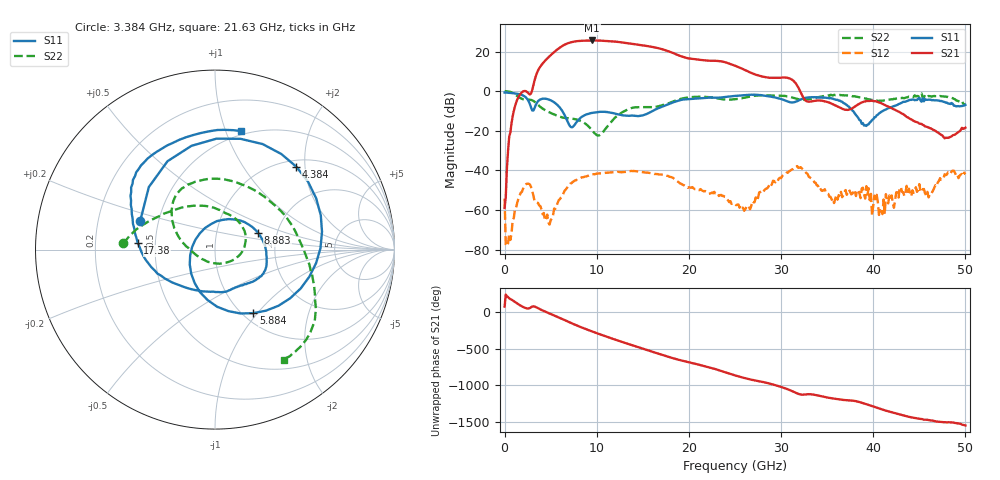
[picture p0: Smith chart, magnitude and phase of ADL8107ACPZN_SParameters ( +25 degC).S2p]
! Analog Devices, Inc.
! Device:	ADL8107ACPZN
! Description:	"GaAs, pHEMT, MMIC, Low Phase Noise Amplifier, 6 GHz to 18 GHz"
! Conditions:	Vdd = 5.0 V
!		IDQ = 90 mA quiescent (Self-biased mode)
!		Pin = -20 dBm
!		Operating Temperature = +25 C (at package bottom)
! Product validation unit SN7 soldered down to Evaluation Board as shown on ADL8107-EVALZ User Guide. Board loss de-embedded from S21 magnitude.  All other RF measurements reference to RF coaxial connector.
! Frequency (GHz)	S11_Mag (dB)	S11_Phase (deg)	S21_Mag (dB)	S21_Phase (deg)	S12_Mag (dB)	S12_Phase (deg)	S22_Mag (dB)	S22_Phase (deg)
#  GHZ  S  DB  R 50
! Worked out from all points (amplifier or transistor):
!   401 points, 10 MHz to 50 GHz, reference 50 ohm
!   highest |S21| = 25.6 dB at 9.508 GHz (marker M1)
!   |S21| within 3 dB of that: 6.202 GHz to 15.71 GHz (9.505 GHz wide, 86.8 % of centre)
!   unconditionally stable (mu >= 1): 65.49 MHz to end of sweep
!   at 8.258 GHz: K = 3.88, MAG = 25.8 dB, |S12| = -43.8 dB
!   at 25.01 GHz: K = 20.05, MAG = 18.8 dB, |S12| = -56.8 dB
!   at 50 GHz: K = 330.01, MAG = -16.5 dB, |S12| = -41.9 dB
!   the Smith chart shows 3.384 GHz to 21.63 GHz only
!   S11 on the Smith chart (normalised r, x): 3.384 GHz: 0.39, +0.16; 4.384 GHz: 1.14, +1.80; 5.884 GHz: 1.11, -0.95; 8.883 GHz: 1.60, +0.32; 17.38 GHz: 0.40, +0.04; 21.63 GHz: 0.46, +1.13
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0.01  -0.71 179.9  -59.03 79.2  -54.23 161.1  0.01 -0.7
3.384325  -7.01 159.2  7.45 73.8  -56.05 -37.3  -5.82 176.0
4.384125  -3.78 45.5  15.28 12.1  -65.29 -42.4  -9.56 141.1
5.883825  -7.67 -58.9  21.59 -68.9  -54.93 41.4  -12.65 91.2
6.883625  -15.76 -149.7  24.20 -126.3  -48.08 14.5  -13.60 61.5
7.633475  -16.85 98.9  25.09 -168.0  -45.10 -15.3  -14.14 36.5
8.383325  -12.96 43.0  25.44 153.1  -43.52 -41.2  -15.38 10.4
8.883225  -11.75 21.0  25.54 128.7  -43.04 -58.4  -16.78 -9.4
9.5081  -10.98 0.7  25.59 98.9  -41.98 -77.4  -19.80 -42.0
10.38292  -10.42 -18.0  25.51 58.6  -41.53 -106.2  -21.98 -123.0
11.5077  -10.86 -34.5  25.21 8.9  -41.02 -141.9  -15.83 173.4
13.5073  -12.44 -66.0  24.17 -75.3  -40.49 159.2  -8.97 130.8
15.25695  -11.83 -120.0  22.94 -146.4  -41.08 100.8  -8.07 85.4
16.75665  -8.46 -167.8  21.61 152.6  -42.11 54.6  -7.56 34.1
17.38153  -7.29 175.1  20.78 127.5  -42.30 34.5  -6.75 12.4
19.13117  -4.43 139.5  17.66 63.8  -46.69 -22.2  -3.87 -29.0
21.63067  -3.40 77.8  15.63 -13.2  -50.61 -65.0  -2.80 -57.8
25.005  -2.39 -46.0  12.84 -141.9  -56.77 -114.2  -4.08 -147.9
28.62927  -2.58 -127.4  6.85 110.4  -48.27 -128.9  -2.15 158.6
33.37832  -3.03 72.1  -5.11 -42.2  -44.82 -30.4  -3.75 29.3
41.75165  -8.48 -118.8  -8.04 82.4  -52.68 -141.3  -4.24 -98.2
50  -6.92 14.4  -18.45 -106.8  -41.91 41.1  -6.87 146.3
